(* Logix 5000 AddOnInstructionDefinition export Banner_K50ProL2_PD_v4; software revision 33.00 *)

TYPE Banner_K50ProL2_PDO_v4 :   // UDT that records the converted prcoess data.
STRUCT
   Reserved : SINT;   // Reserved
   Color_2_Intensity : SINT;   // 0=high, 1=low, 2=medium, 3=custom, 4=off
   Color_1_Intensity : SINT;   // 0=high, 1=low, 2=medium, 3=custom, 4=off
   Animation_Type : SINT;   // 0=off, 1=steady, 2=flash,3=two color flash, 4=strobe, 5=half/half, 6=half/half rotate, 7=chase, 8=demo mode
   Rotation_Direction : SINT;   // false=counter clockwise, true=clockwise
   Audible_Mode : SINT;   // 0=off, 1=on, 2=pulse
   Color_2 : SINT;   // 0=green, 1=red, 2=orange, 3=yellow, 4=lime, 5=spring green, 6=cyan, 7=sky blue, 8=blue, 9=violet, 10=magenta, 11=rose, 12=white, 13=custom1, 14=custom2, 15=custom3, 16=custom4, 17=custom5
   Color_Flash_Rate : SINT;   // Hz. 0=1.5, 1=.5, 2=3, 3=6, 4=9, 5=12, 6=Custom
   Color_1 : SINT;   // 0=green, 1=red, 2=orange, 3=yellow, 4=lime, 5=spring green, 6=cyan, 7=sky blue, 8=blue, 9=violet, 10=magenta, 11=rose, 12=white, 13=custom1, 14=custom2, 15=custom3, 16=custom4, 17=custom5
   PDO_DT : SINT[4];
END_STRUCT
END_TYPE

ADD_ON_INSTRUCTION Banner_K50ProL2_PD_v4   (* revision 4.0, vendor Banner Engineering *)
// AOI that controls the state of the K50 Pro L2 Light and Audible Segments.
VAR_IN_OUT
   Process_Data : Banner_K50ProL2_PDO_v4; {required}
END_VAR
VAR_INPUT
   Byte_Swap : BOOL; {required}
END_VAR
VAR
   Temp_Byte_Array : SINT[4]; {access None}
END_VAR

ROUTINE Logic   (* ladder *)
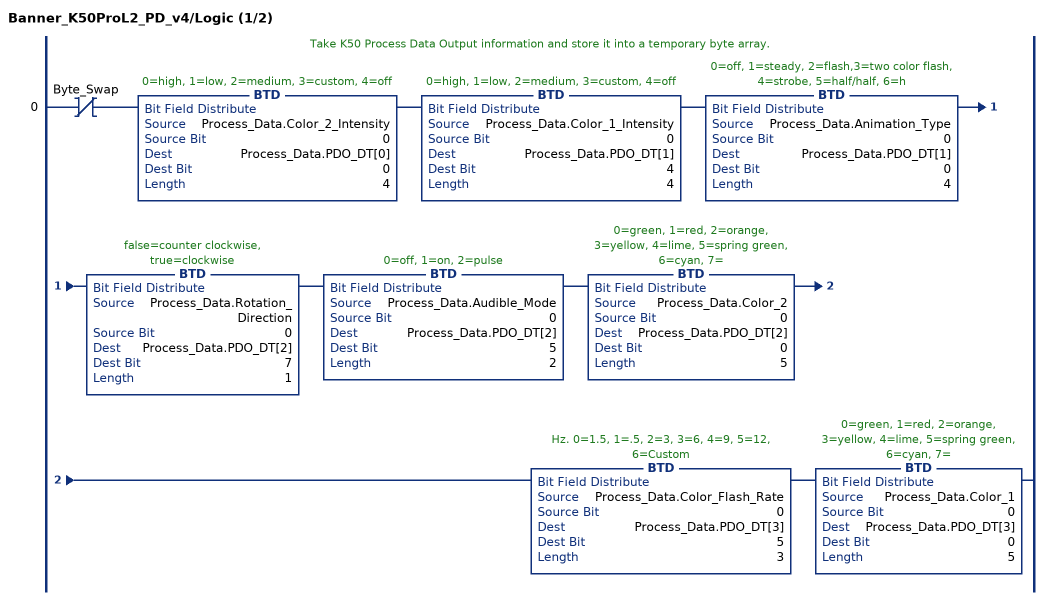
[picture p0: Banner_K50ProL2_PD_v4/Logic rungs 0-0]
   // Take K50 Process Data Output information and store it into a temporary byte array.
   0: XIO(Byte_Swap)BTD(Process_Data.Color_2_Intensity,0,Process_Data.PDO_DT[0],0,4)BTD(Process_Data.Color_1_Intensity,0,Process_Data.PDO_DT[1],4,4)BTD(Process_Data.Animation_Type,0,Process_Data.PDO_DT[1],0,4)BTD(Process_Data.Rotation_Direction,0,Process_Data.PDO_DT[2],7,1)BTD(Process_Data.Audible_Mode,0,Process_Data.PDO_DT[2],5,2)BTD(Process_Data.Color_2,0,Process_Data.PDO_DT[2],0,5)BTD(Process_Data.Color_Flash_Rate,0,Process_Data.PDO_DT[3],5,3)BTD(Process_Data.Color_1,0,Process_Data.PDO_DT[3],0,5);
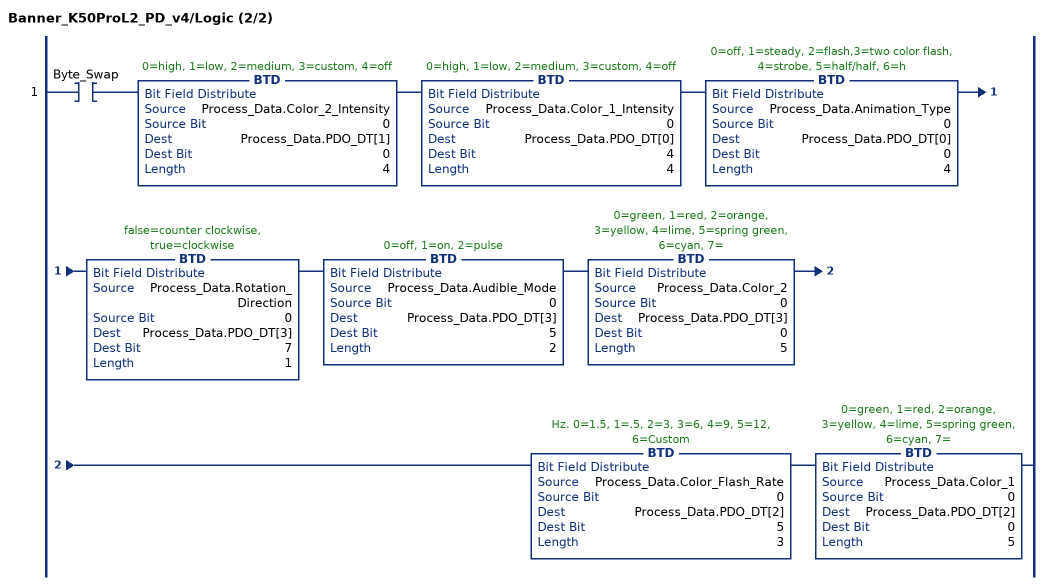
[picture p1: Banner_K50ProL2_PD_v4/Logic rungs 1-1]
   1: XIC(Byte_Swap)BTD(Process_Data.Color_2_Intensity,0,Process_Data.PDO_DT[1],0,4)BTD(Process_Data.Color_1_Intensity,0,Process_Data.PDO_DT[0],4,4)BTD(Process_Data.Animation_Type,0,Process_Data.PDO_DT[0],0,4)BTD(Process_Data.Rotation_Direction,0,Process_Data.PDO_DT[3],7,1)BTD(Process_Data.Audible_Mode,0,Process_Data.PDO_DT[3],5,2)BTD(Process_Data.Color_2,0,Process_Data.PDO_DT[3],0,5)BTD(Process_Data.Color_Flash_Rate,0,Process_Data.PDO_DT[2],5,3)BTD(Process_Data.Color_1,0,Process_Data.PDO_DT[2],0,5);
END_ROUTINE
END_ADD_ON_INSTRUCTION
